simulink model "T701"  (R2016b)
settings: Solver=VariableStepAuto  StartTime=0.0  StopTime=612  RelTol=1e-3
libraries: simulink x6, sldrtlib x1

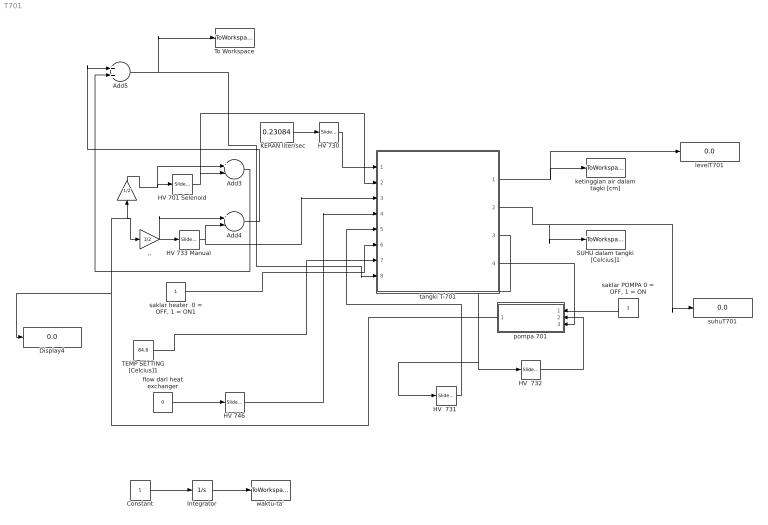
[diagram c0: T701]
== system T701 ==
  ,. : Gain  RequirementInfo={} %GIDa_190d4ec9_c50e_4f69_aeb1_9cdf85c6f1c6  Gain=1/2
  .. : Gain  RequirementInfo={} %GIDa_7c5a45c1_d067_497b_821d_d880dc9dc83c  Gain=1/2
  Add3 : Sum  RequirementInfo={} %GIDa_1bf521dd_8915_4687_9355_da1ce3a05a06  Inputs=+-
  Add4 : Sum  RequirementInfo={} %GIDa_6b78beb4_9619_4fad_b40d_0695c7aad7a1  Inputs=+-
  Add5 : Sum  RequirementInfo={} %GIDa_9296d099_40b6_4b83_9ef9_f383de4b6f71
  Constant : Constant  RequirementInfo={} %GIDa_a44811d7_9bc1_4eb1_8796_a12e2adcf7f3
  Display4 : Display
  "HV  731 " : simulink/Math Operations/Slider Gain  low=0  gain=0  high=1
  HV  732 : simulink/Math Operations/Slider Gain  low=0  gain=0  high=1
  HV 701 Selenoid : simulink/Math Operations/Slider Gain  low=0  gain=0  high=1
  HV 730 : simulink/Math Operations/Slider Gain  low=0  gain=0  high=1
  HV 733 Manual : simulink/Math Operations/Slider Gain  low=0  gain=0  high=1
  HV 746 : simulink/Math Operations/Slider Gain  low=0  gain=0  high=1
  Integrator : Integrator  RequirementInfo={} %GIDa_5f0a8732_fad7_40fd_b198_912f63833c27
  KERAN liter/sec : Constant  RequirementInfo={} %GIDa_88508e06_78e5_426b_90d6_5d8dbfa59593  Value=0.23084
  SUHU dalam tangki [Celcius]1 : ToWorkspace  VariableName=suhuT701  SampleTime=-1
  TEMP SETTING [Celcius]1 : Constant  RequirementInfo={} %GIDa_3a60333b_7f9f_49e1_89b6_c26a2249b7cd  Value=84.8
  To Workspace : ToWorkspace  VariableName=flowF705  SaveFormat=Timeseries  SampleTime=-1
  flow dari heat exchanger : Constant  RequirementInfo={} %GIDa_b8b485b4_8e51_4aad_843f_87516184033e  Value=0
  ketinggian air dalam tagki [cm] : ToWorkspace  VariableName=levelT701  SampleTime=-1
  levelT701 : Display
  pompa 701 : Subsystem  RequirementInfo={} %GIDa_cf73bed5_9f1a_4afd_9371_96a52dea213c
  "saklar heater  0 = OFF, 1 = ON1" : Constant  RequirementInfo={} %GIDa_6bdf1fa7_d8e5_4ff9_a893_45fa27124c37
  "saklar POMPA 0 = OFF, 1 = ON" : Constant  RequirementInfo={} %GIDa_da1bea97_cc50_45e0_b3ff_ae5b97cd4c07
  suhuT701 : Display
  tangki T-701 : Subsystem  RequirementInfo={} %GIDa_363135a2_d77c_4695_bcec_bcc033992816
  waktu-ta' : ToWorkspace  VariableName=time  SampleTime=-1
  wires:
  tangki T-701/1(level [cm]) -> ketinggian air dalam tagki [cm]/1, levelT701/1
  HV 730/1 -> tangki T-701/1(In1)
  KERAN liter/sec/1 -> HV 730/1
  HV 746/1 -> tangki T-701/4(In4)
  pompa 701/1(Out1) -> ,./1, ../1, Display4/1
  "saklar POMPA 0 = OFF, 1 = ON"/1 -> pompa 701/1(saklar remote)
  tangki T-701/3(debit out (Liter/sec)) -> "HV  731 "/1, HV  732/1
  "HV  731 "/1 -> tangki T-701/5(In6)
  TEMP SETTING [Celcius]1/1 -> tangki T-701/7(setting)
  HV 733 Manual/1 -> tangki T-701/3(In3), Add4/2
  HV 701 Selenoid/1 -> tangki T-701/2(In2), Add3/2
  Add3/1 -> Add5/2
  Add4/1 -> Add5/1
  ../1 -> Add3/1, HV 701 Selenoid/1
  ,./1 -> Add4/1, HV 733 Manual/1
  tangki T-701/4(to pompa) -> pompa 701/3(LSL 701)
  HV  732/1 -> pompa 701/2(In2)
  tangki T-701/2(suhu [Celcius]) -> SUHU dalam tangki [Celcius]1/1, suhuT701/1
  flow dari heat exchanger/1 -> HV 746/1
  "saklar heater  0 = OFF, 1 = ON1"/1 -> tangki T-701/6(remote on/off)
  Add5/1 -> To Workspace/1, tangki T-701/8(In7)
  Constant/1 -> Integrator/1
  Integrator/1 -> waktu-ta'/1

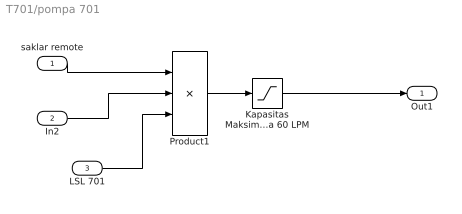
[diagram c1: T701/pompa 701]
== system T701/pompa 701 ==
  saklar remote : Inport  RequirementInfo={} %GIDa_dc5fee78_314e_4645_bffd_89647433657e
  In2 : Inport  RequirementInfo={} %GIDa_18e5cee8_f883_440b_99da_9359bc48fe03  Port=2
  LSL 701 : Inport  RequirementInfo={} %GIDa_765d9484_7740_4d48_b52e_3d89d31f8db0  Port=3
  Kapasitas Maksimum Pompa 60 LPM : Saturate  RequirementInfo={} %GIDa_66a4c416_9289_4217_afbb_96d7b6c06c39  UpperLimit=1  LowerLimit=0  LinearizeAsGain=off  ZeroCross=off
  Product1 : Product  RequirementInfo={} %GIDa_4798ad51_5846_4fbe_a128_22b0c00c6bcc  Inputs=3
  Out1 : Outport  RequirementInfo={} %GIDa_b489e170_cc79_4854_bc2b_87b8b4dd23b0
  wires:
  Kapasitas Maksimum Pompa 60 LPM/1 -> Out1/1
  Product1/1 -> Kapasitas Maksimum Pompa 60 LPM/1
  LSL 701/1 -> Product1/3
  In2/1 -> Product1/2
  saklar remote/1 -> Product1/1

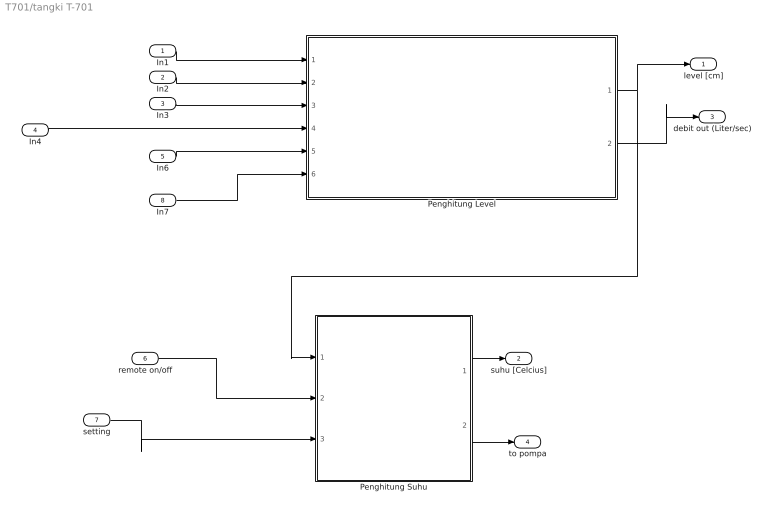
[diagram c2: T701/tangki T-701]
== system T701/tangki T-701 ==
  In1 : Inport  RequirementInfo={} %GIDa_eb5444c4_72cd_4788_a83f_d59f1c90e647
  In2 : Inport  RequirementInfo={} %GIDa_08951b4a_c586_4e30_9528_8ea22dd783b8  Port=2
  In3 : Inport  RequirementInfo={} %GIDa_a7c50569_9a58_4fd7_9621_b1438c5f35f0  Port=3
  In4 : Inport  RequirementInfo={} %GIDa_7b220f4c_5455_4a45_84a1_b44681cc8b9b  Port=4
  In6 : Inport  RequirementInfo={} %GIDa_7d9e6876_2322_4fc0_a972_8b63c1ec7f9f  Port=5
  remote on/off : Inport  RequirementInfo={} %GIDa_68c38f9f_d4f2_4654_97c2_3f42f565a059  Port=6
  setting : Inport  RequirementInfo={} %GIDa_d5ef20cc_fc81_4d60_99e7_7b4ac428f7b5  Port=7
  In7 : Inport  RequirementInfo={} %GIDa_ca280e05_3d3c_4bdb_b2e0_d3ec9ecc32b0  Port=8
  Penghitung Level : Subsystem  RequirementInfo={} %GIDa_7ab81b33_5e10_4fd7_a909_a5376bb0157f
  Penghitung Suhu : Subsystem  RequirementInfo={} %GIDa_272349a2_2a45_4fac_8380_fd2221c6883f
  level [cm] : Outport  RequirementInfo={} %GIDa_d6658841_302c_4627_80ea_690171a444ca
  suhu [Celcius] : Outport  RequirementInfo={} %GIDa_4c3fd961_0ce9_4aa9_a394_fa5f0ceee7a0  Port=2
  debit out (Liter/sec) : Outport  RequirementInfo={} %GIDa_38c8d8f4_932f_4d4b_9064_98a84cd529e5  Port=3
  to pompa : Outport  RequirementInfo={} %GIDa_ce821ec2_649a_454b_a138_3ca7cb117957  Port=4
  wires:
  In1/1 -> Penghitung Level/1(dari keran via HV-730)
  In2/1 -> Penghitung Level/2(Dari Pompa lewat HV-701)
  In3/1 -> Penghitung Level/3(Dari Pompa lewat HV-733)
  In6/1 -> Penghitung Level/5(Drain)
  In7/1 -> Penghitung Level/6(HV 732 ke Pompa)
  Penghitung Level/2(debit out (Liter/sec)) -> debit out (Liter/sec)/1
  Penghitung Level/1(level [cm]) -> level [cm]/1, Penghitung Suhu/1(level[cm])
  Penghitung Suhu/1(suhu) -> suhu [Celcius]/1
  remote on/off/1 -> Penghitung Suhu/2(Remote Heater)
  In4/1 -> Penghitung Level/4(Dari Heat-Exc  lewat HV-746)
  setting/1 -> Penghitung Suhu/3(Set Point)
  Penghitung Suhu/2(to pompa) -> to pompa/1

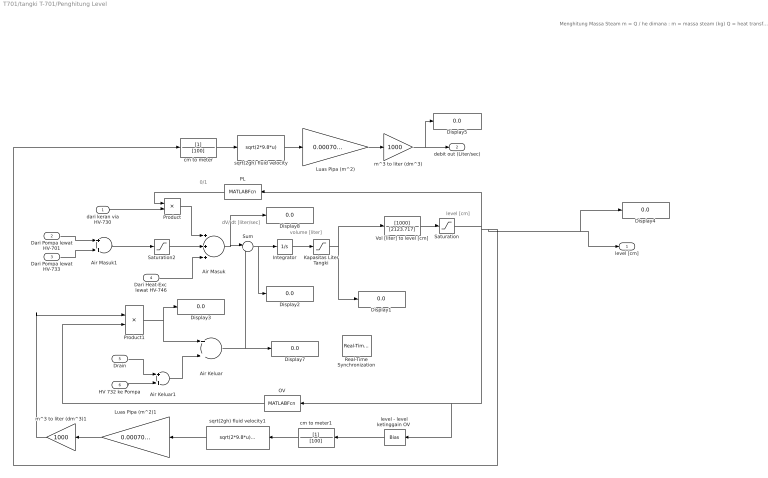
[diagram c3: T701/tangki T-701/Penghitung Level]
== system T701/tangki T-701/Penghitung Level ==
  note: 0/1
  note: dV/ dt [liter/sec]
  note: level [cm]
  note: volume [liter]
  note: Menghitung Massa Steam m = Q / he dimana : m = massa steam (kg) Q = heat transfer (J) he = Spesific laten heat evaporation (J/kg)
  dari keran via HV-730 : Inport  RequirementInfo={} %GIDa_b3ca337d_0b00_4c51_af35_2f18d27babd4
  Dari Pompa lewat HV-701 : Inport  RequirementInfo={} %GIDa_23aa178c_5e5a_48ef_b1da_8d682856c4f1  Port=2
  Dari Pompa lewat HV-733 : Inport  RequirementInfo={} %GIDa_fe169ab1_21d3_4959_9277_9c1db7803f78  Port=3
  Dari Heat-Exc  lewat HV-746 : Inport  RequirementInfo={} %GIDa_3f16255f_4c24_42b7_b267_52a44afee3ed  Port=4
  Drain : Inport  RequirementInfo={} %GIDa_c5531827_0415_4b3c_b40a_2151ed12135b  Port=5
  HV 732 ke Pompa : Inport  RequirementInfo={} %GIDa_d3625b86_5728_45ee_93d8_34cc72ef8e32  Port=6
  Air Keluar : Sum  RequirementInfo={} %GIDa_901fff7c_1227_4ccc_9f52_ce661dd58fb0
  Air Keluar1 : Sum  RequirementInfo={} %GIDa_4e7036a1_e4d9_461c_aa1e_581360c4e0ae
  Air Masuk : Sum  RequirementInfo={} %GIDa_4a40ff64_8362_4ec0_9947_ce173dfa37c4  Inputs=+++
  Air Masuk1 : Sum  RequirementInfo={} %GIDa_41cef2aa_10c6_4b2c_930a_455844505c60
  Display{1..5,7..8} (7 alike) : Display
  Integrator : Integrator  RequirementInfo={} %GIDa_272909bc_6e08_42b5_8925_3792f57c92cc
  Kapasitas Liter Tangki : Saturate  RequirementInfo={} %GIDa_f98a18e0_925c_4287_b88a_530af3b2c562  UpperLimit=120  LowerLimit=-99999999999999999999999999999999999999999999999999999999
  Luas Pipa (m^2) : Gain  RequirementInfo={} %GIDa_4166dbfe_27aa_4a90_95fd_ba265bc6a1ac  Gain=0.000706858347
  Luas Pipa (m^2)1 : Gain  RequirementInfo={} %GIDa_21f5673e_1fe2_4c83_b020_3ecdb6cd9c6a  Gain=0.000706858347
  OV : MATLABFcn  RequirementInfo={} %GIDa_bc2e0a84_e429_41f7_83cd_87442e39be95  MATLABFcn=OV
  PL : MATLABFcn  RequirementInfo={} %GIDa_3ef59baa_c373_494b_bbbf_9dd7865ddc54  MATLABFcn=PL
  Product : Product  RequirementInfo={} %GIDa_4c1da06b_3117_45da_a7fb_1b94b3542d54
  Product1 : Product  RequirementInfo={} %GIDa_d3c5aae6_351a_4e0d_b0dc_c62be6ed28d4
  Real-Time Synchronization : sldrtlib/Real-Time Synchronization  SampleTime=0.1  MaxMissedTicks=10  ShowMissedTicks=off  YieldWhenWaiting=off
  Saturation : Saturate  RequirementInfo={} %GIDa_135c984c_fc92_4729_a7d9_22191eb5a4b6  UpperLimit=65.5  LowerLimit=0
  Saturation2 : Saturate  RequirementInfo={} %GIDa_a4699b6b_5582_4c70_bf49_ec5c84ab5ff2  UpperLimit=1  LowerLimit=-999999999999999999999999999999999999999999999999999999
  Sum : Sum  RequirementInfo={} %GIDa_6300aad4_3ab8_4103_b18b_d1830c35d826  Inputs=|+-
  Vol [liter] to level [cm] : TransferFcn  RequirementInfo={} %GIDa_f18758fb_2b1a_4ca4_b583_20eedb98c198  Numerator=[1000]  Denominator=[2123.717]
  cm to meter : TransferFcn  RequirementInfo={} %GIDa_c0850802_b9af_4be1_8877_a68cbd9dcff3  Denominator=[100]
  cm to meter1 : TransferFcn  RequirementInfo={} %GIDa_efa7640e_0f65_4f02_ae67_b13020d97b27  Denominator=[100]
  "level - level ketinggain OV " : Bias  RequirementInfo={} %GIDa_43ef5038_2f80_4a7f_acb5_b9104beca26f  Bias=-60
  m^3 to liter (dm^3) : Gain  RequirementInfo={} %GIDa_efd887bb_44a5_4228_b2d7_98cd84856196  Gain=1000
  m^3 to liter (dm^3)1 : Gain  RequirementInfo={} %GIDa_d27a5346_4a9a_447c_9c53_c697b5752e3e  Gain=1000
  sqrt(2gh) fluid velocity : Fcn  RequirementInfo={} %GIDa_dbad9609_718e_46b2_a0fd_d620594525d9  Expr=sqrt(2*9.8*u)
  sqrt(2gh) fluid velocity1 : Fcn  RequirementInfo={} %GIDa_e35ec909_4b47_4125_99c7_9fcc0c597732  Expr=sqrt(2*9.8*u)+0.00001
  level [cm] : Outport  RequirementInfo={} %GIDa_af6b1aea_e9c3_47eb_8e83_29db6a6d47b2
  debit out (Liter/sec) : Outport  RequirementInfo={} %GIDa_84a53a7f_12da_44b5_8630_e91dd5789c7e  Port=2
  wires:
  Vol [liter] to level [cm]/1 -> Saturation/1
  Integrator/1 -> Kapasitas Liter Tangki/1
  Sum/1 -> Integrator/1, Display2/1
  Air Masuk/1 -> Display8/1, Sum/1
  Dari Heat-Exc  lewat HV-746/1 -> Air Masuk/3
  Product/1 -> Air Masuk/1
  dari keran via HV-730/1 -> Product/2
  PL/1 -> Product/1
  m^3 to liter (dm^3)1/1 -> Product1/1
  OV/1 -> Product1/2
  Product1/1 -> Display3/1, Air Keluar/1
  Drain/1 -> Air Keluar1/1
  HV 732 ke Pompa/1 -> Air Keluar1/2
  Air Keluar1/1 -> Air Keluar/2
  Air Keluar/1 -> Display7/1, Sum/2
  m^3 to liter (dm^3)/1 -> Display5/1, debit out (Liter/sec)/1
  sqrt(2gh) fluid velocity/1 -> Luas Pipa (m^2)/1
  Luas Pipa (m^2)/1 -> m^3 to liter (dm^3)/1
  cm to meter/1 -> sqrt(2gh) fluid velocity/1
  cm to meter1/1 -> sqrt(2gh) fluid velocity1/1
  sqrt(2gh) fluid velocity1/1 -> Luas Pipa (m^2)1/1
  Luas Pipa (m^2)1/1 -> m^3 to liter (dm^3)1/1
  "level - level ketinggain OV "/1 -> cm to meter1/1
  Dari Pompa lewat HV-733/1 -> Air Masuk1/2
  Dari Pompa lewat HV-701/1 -> Air Masuk1/1
  Air Masuk1/1 -> Saturation2/1
  Saturation2/1 -> Air Masuk/2
  Kapasitas Liter Tangki/1 -> Vol [liter] to level [cm]/1, Display1/1
  Saturation/1 -> "level - level ketinggain OV "/1, OV/1, Display4/1, level [cm]/1, cm to meter/1, PL/1

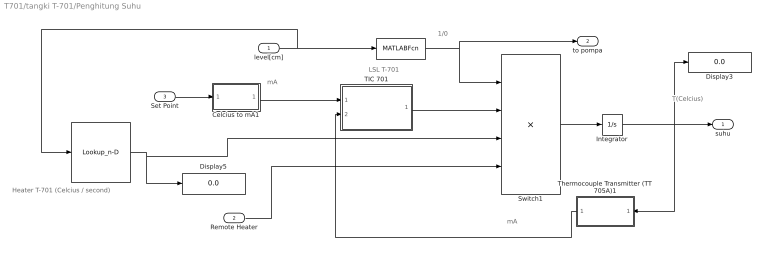
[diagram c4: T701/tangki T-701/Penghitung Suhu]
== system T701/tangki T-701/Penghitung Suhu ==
  note: Heater T-701 (Celcius / second)
  note: mA
  note: mA
  note: T(Celcius)
  note: LSL T-701
  note: 1/0
  level[cm] : Inport  RequirementInfo={} %GIDa_9ba8d1f3_b6d5_4e86_9b5f_7bc8b27dc16d
  Remote Heater : Inport  RequirementInfo={} %GIDa_2e4e6060_e341_4fbc_ae1f_fd5f29a0ae63  Port=2
  Set Point : Inport  RequirementInfo={} %GIDa_65ae9324_91a4_4306_bc74_a1da1ab60f8b  Port=3
  " " : MATLABFcn  RequirementInfo="{'linktype_rmi_simulink' 'D' ':376' 'true' 'D/Lamp  (SubSystem)' '' } %GIDa_7afa07d7_9cfc_4111_b913_e6631543cbd9"  MATLABFcn=LSL
  . : Lookup_n-D  NumberOfTableDimensions=1  BreakpointsForDimension1=[30,40,50]  Table=[0.068311,0.054088,0.042156]  InternalRulePriority=Speed  RndMeth=Simplest
  Celcius to mA1 : Subsystem  RequirementInfo={} %GIDa_8bbf1dbc_2c30_4270_b4bf_9a03daf9ae7f
  Display3 : Display
  Display5 : Display
  Integrator : Integrator  RequirementInfo={} %GIDa_4b0ca7b8_1c08_4880_aa15_ba4c6b8c015d  InitialCondition=32.2
  Switch1 : Product  RequirementInfo={} %GIDa_6f9abdb3_76d5_48c8_9c4a_d44b38f35c97  Inputs=4
  TIC 701 : Subsystem  RequirementInfo={} %GIDa_bdd29add_fa85_4c6e_98b1_1a1f9a3f6249
  Thermocouple Transmitter (TT 705A)1 : Subsystem  RequirementInfo={} %GIDa_7e8bc1fe_ae87_481a_bab6_07e08e89235b
  suhu : Outport  RequirementInfo={} %GIDa_caae0911_dd84_4a4f_b2ce_8ed43bb16568
  to pompa : Outport  RequirementInfo={} %GIDa_d1665a25_0e79_49f2_b0f2_3c47f5c55ad9  Port=2
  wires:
  Switch1/1 -> Integrator/1
  Remote Heater/1 -> Switch1/4
  TIC 701/1(Out1) -> Switch1/2
  " "/1 -> Switch1/1, to pompa/1
  ./1 -> Display5/1, Switch1/3
  Thermocouple Transmitter (TT 705A)1/1(Out1) -> TIC 701/2(In2)
  Set Point/1 -> Celcius to mA1/1(In1)
  Celcius to mA1/1(Out1) -> TIC 701/1(In1)
  Integrator/1 -> Thermocouple Transmitter (TT 705A)1/1(In1), suhu/1, Display3/1
  level[cm]/1 -> ./1, " "/1

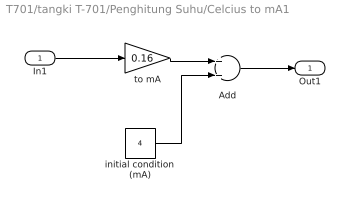
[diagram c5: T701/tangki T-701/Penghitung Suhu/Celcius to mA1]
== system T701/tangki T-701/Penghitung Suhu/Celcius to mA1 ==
  In1 : Inport  RequirementInfo={} %GIDa_1e57a378_666d_412e_8f0c_3f8aaa42362b
  Add : Sum  RequirementInfo={} %GIDa_4fe5a67a_1c8f_4803_8c00_ce2ffc86e1a7
  initial condition (mA) : Constant  RequirementInfo={} %GIDa_0a816788_5d74_4fc6_9be3_a818e7d3613c  Value=4
  to mA : Gain  RequirementInfo={} %GIDa_45ff5a7d_c6b9_45df_879b_4e17107c08b7  Gain=0.16
  Out1 : Outport  RequirementInfo={} %GIDa_b8063ecc_200d_421b_b0f0_e8f5666ea5aa
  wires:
  In1/1 -> to mA/1
  to mA/1 -> Add/1
  Add/1 -> Out1/1
  initial condition (mA)/1 -> Add/2

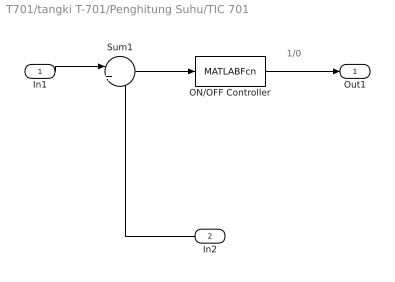
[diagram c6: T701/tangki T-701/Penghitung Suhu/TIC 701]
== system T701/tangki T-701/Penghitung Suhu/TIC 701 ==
  note: 1/0
  In1 : Inport  RequirementInfo={} %GIDa_60ee68c3_1040_412e_a9a9_b5f8e8a2e603
  In2 : Inport  RequirementInfo={} %GIDa_eef0fa26_5ab4_4940_8ac3_a1093278cd07  Port=2
  ON/OFF Controller : MATLABFcn  RequirementInfo={} %GIDa_68d0746f_709f_44a1_bccd_7313d62453b0  MATLABFcn=TM
  Sum1 : Sum  RequirementInfo={} %GIDa_e330533b_0273_4f08_b914_c37355adb3f5  Inputs=|+-
  Out1 : Outport  RequirementInfo={} %GIDa_e9617866_45b0_4bbb_8b6c_eb5d99552921
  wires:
  In2/1 -> Sum1/2
  Sum1/1 -> ON/OFF Controller/1
  In1/1 -> Sum1/1
  ON/OFF Controller/1 -> Out1/1

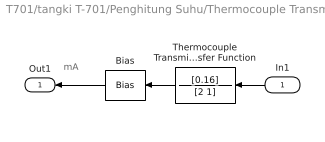
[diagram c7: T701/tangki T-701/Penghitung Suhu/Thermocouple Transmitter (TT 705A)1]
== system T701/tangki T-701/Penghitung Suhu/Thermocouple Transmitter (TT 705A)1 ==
  note: mA
  In1 : Inport  RequirementInfo={} %GIDa_0e9006b7_ab38_4005_8a19_9e8a7982983a
  Bias : Bias  RequirementInfo={} %GIDa_ad44890e_d02d_4be8_b9dd_8a75286ee440  Bias=4
  Thermocouple Transmitter Transfer Function : TransferFcn  RequirementInfo={} %GIDa_f1c7a1a4_5076_491e_a860_3be442c80425  Numerator=[0.16]  Denominator=[2 1]
  Out1 : Outport  RequirementInfo={} %GIDa_64d7d141_c903_45a4_8bed_4c2f0bbe590a
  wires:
  Bias/1 -> Out1/1
  In1/1 -> Thermocouple Transmitter Transfer Function/1
  Thermocouple Transmitter Transfer Function/1 -> Bias/1
